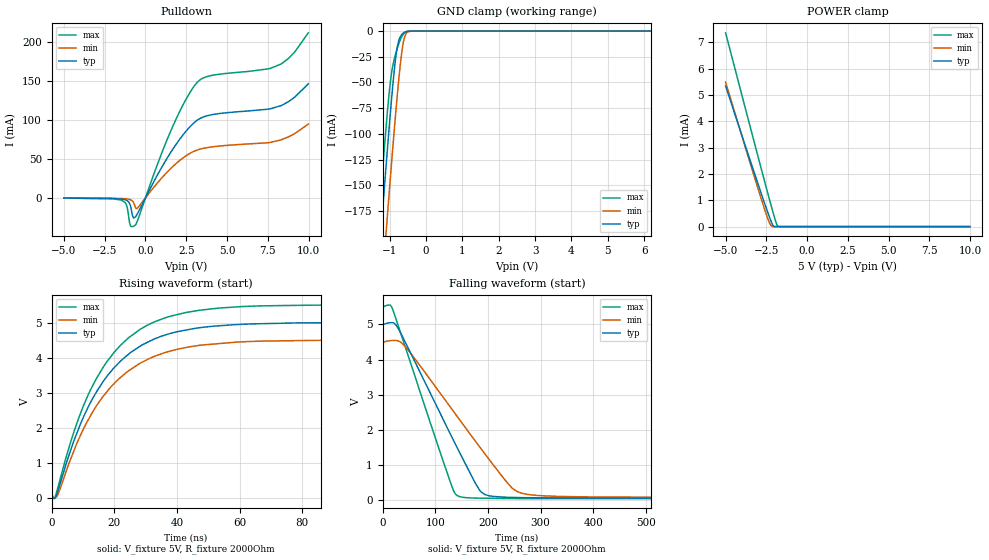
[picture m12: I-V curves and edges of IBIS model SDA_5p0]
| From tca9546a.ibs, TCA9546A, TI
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|   Model
[Model]   SDA_5p0
Model_type   I/O_open_drain
Polarity   Non-Inverting
Enable   Active-Low
Vinl = 1.5
Vinh = 3.5
Vmeas = 2.5
Vref = 5
Cref = 1pF
Rref = 2000
|   typ   min   max
C_comp   3.666pF   3.611pF   3.839pF
[Voltage Range]   5   4.5   5.5
[Temperature Range]   27   125   -40
[Pullup Reference]   5   4.5   5.5
[Pulldown Reference]   -0   -0   -0
[Power Clamp Reference]   5   4.5   5.5
[GND Clamp Reference]   -0   -0   -0
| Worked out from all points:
|   slope of the pulldown table from 0 to 0.75 V, typ, clamps not added: 24.9 ohm
|   GND clamp passes 1 mA (typ) near -0.58 V on its own axis
|   POWER clamp passes 1 mA (typ) near -2.67 V on its own axis
|   falling waveform, V_fixture 5V, R_fixture 2000Ohm: 20-80 % time 97.7ns typ, 131ns min, 72.4ns max; typ from 5 V to 0.059 V
|   rising waveform, V_fixture 5V, R_fixture 2000Ohm: 20-80 % time 18.5ns typ, 19ns min, 18.2ns max; typ from 0.059 V to 5 V
[Pulldown]
|   Voltage   I(typ)   I(min)   I(max)
-5V       -210.1uA   -127.1uA   -293.9uA
-1.49V    -1.489mA   -739.4uA   -2.775mA
-1.175V   -2.989mA   -1.22mA    -8.529mA
-1.025V   -5.347mA   -1.731mA   -24.71mA
-920mV    -10.07mA   -2.398mA   -35.99mA
-725mV    -25.8mA    -6.186mA   -36.45mA
-485mV    -19.98mA   -13.01mA   -29.06mA
1.69V     63.1mA     40.62mA    92.74mA
3.16V     99.78mA    61.5mA     148.4mA
4V        106.7mA    65.4mA     157.3mA
8.305V    118.7mA    74.68mA    172.2mA
9.985V    146.8mA    95mA       212.4mA
[GND Clamp]
|   Voltage   I(typ)   I(min)   I(max)
-5V       -2.043A    -2.104A    -2.005A
-1.43V    -284mA     -349.8mA   -243.2mA
-1.25V    -199mA     -264.7mA   -158.8mA
-1.235V   -192mA     -257.7mA   -151.9mA
-1.13V    -143.7mA   -208.9mA   -105.1mA
-1.085V   -123.4mA   -188.2mA   -86.17mA
-980mV    -77.94mA   -140.9mA   -48.34mA
-875mV    -37.65mA   -95.34mA   -27mA
-815mV    -20.17mA   -70.71mA   -19.2mA
-680mV    -3.857mA   -23.41mA   -6.177mA
-560mV    -645.4uA   -2.929mA   -964.8uA
9.985V    0A         0A         0A
[POWER Clamp]
|   Voltage   I(typ)   I(min)   I(max)
-5V       5.337mA    5.487mA    7.358mA
-3.155V   1.886mA    1.729mA    2.998mA
-2.435V   577.6uA    345.3uA    1.319mA
-2.255V   272.8uA    77.4uA     907.1uA
-2.18V    157.4uA    19.51uA    738uA
-2.09V    46.43uA    1.748uA    538.3uA
-1.91V    23.25nA    0A         165.4uA
-1.805V   0A         0A         18.81uA
9.985V    0A         0A         0A
[Ramp]
R_load = 2000
|   typ   min   max
dV/dt_r   2.96458/1.85497e-08   2.65166/1.90001e-08   3.27326/1.81762e-08
dV/dt_f   2.96459/9.76757e-08   2.65166/1.30752e-07   3.27327/7.24288e-08
[Falling Waveform]
V_fixture = 5V
V_fixture_min = 4.5V
V_fixture_max = 5.5V
R_fixture = 2000Ohm
C_fixture = 0F
|   Time   V(typ)   V(min)   V(max)
0s        5V         4.5V       5.5V
18.4ns    5.05V      4.544V     5.461V
43.66ns   4.479V     4.363V     4.339V
129.5ns   1.863V     2.634V     485.3mV
145.7ns   1.376V     2.301V     106.5mV
177.6ns   447mV      1.654V     60.88mV
193.8ns   164.8mV    1.329V     57.77mV
246ns     80.53mV    344.6mV    49.21mV
273.2ns   73.02mV    171mV      48.1mV
1us       59.02mV    80.54mV    44.55mV
[Rising Waveform]
V_fixture = 5V
V_fixture_min = 4.5V
V_fixture_max = 5.5V
R_fixture = 2000Ohm
C_fixture = 0F
|   Time   V(typ)   V(min)   V(max)
0s        59.02mV    80.54mV    44.55mV
767.5ps   3.873mV    19.31mV    -10.92mV
1.825ns   170.5mV    79.41mV    256.1mV
6.41ns    1.461V     1.198V     1.706V
11.65ns   2.594V     2.228V     2.942V
16.59ns   3.341V     2.916V     3.75V
21.92ns   3.897V     3.433V     4.348V
36.13ns   4.641V     4.144V     5.13V
60.69ns   4.948V     4.45V      5.453V
1us       5V         4.5V       5.5V
